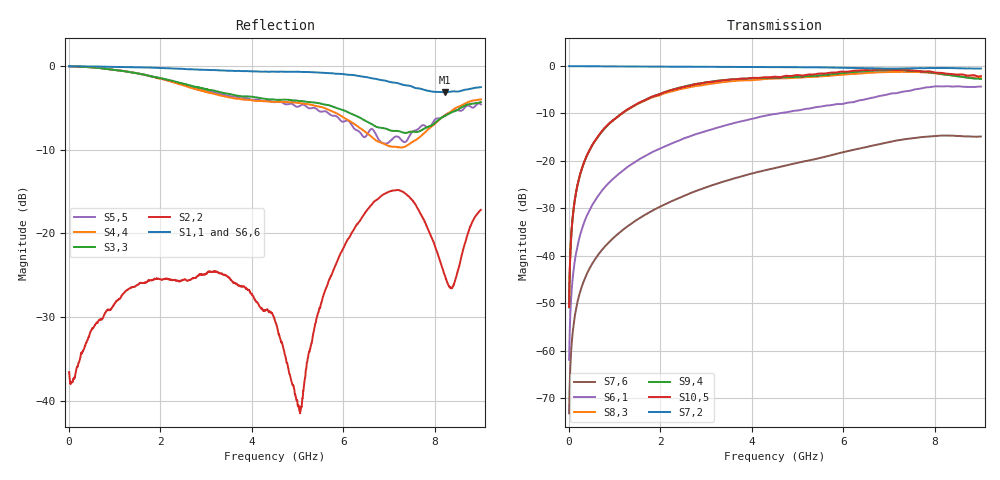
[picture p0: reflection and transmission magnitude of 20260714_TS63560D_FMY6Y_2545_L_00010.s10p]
# GHz S DB R 50
! CMT, SN0916, 25263762, 26.7.0
! Date: 15.07.2026 13:19:08
! Data: Format
! Freq S1.1:dB/Ang S1.2:dB/Ang S1.3:dB/Ang S1.4:dB/Ang S1.5:dB/Ang S1.6:dB/Ang S1.7:dB/Ang S1.8:dB/Ang S1.9:dB/Ang S1.10:dB/Ang
!  S2.1:dB/Ang S2.2:dB/Ang S2.3:dB/Ang S2.4:dB/Ang S2.5:dB/Ang S2.6:dB/Ang S2.7:dB/Ang S2.8:dB/Ang S2.9:dB/Ang S2.10:dB/Ang
!  S3.1:dB/Ang S3.2:dB/Ang S3.3:dB/Ang S3.4:dB/Ang S3.5:dB/Ang S3.6:dB/Ang S3.7:dB/Ang S3.8:dB/Ang S3.9:dB/Ang S3.10:dB/Ang
!  S4.1:dB/Ang S4.2:dB/Ang S4.3:dB/Ang S4.4:dB/Ang S4.5:dB/Ang S4.6:dB/Ang S4.7:dB/Ang S4.8:dB/Ang S4.9:dB/Ang S4.10:dB/Ang
!  S5.1:dB/Ang S5.2:dB/Ang S5.3:dB/Ang S5.4:dB/Ang S5.5:dB/Ang S5.6:dB/Ang S5.7:dB/Ang S5.8:dB/Ang S5.9:dB/Ang S5.10:dB/Ang
!  S6.1:dB/Ang S6.2:dB/Ang S6.3:dB/Ang S6.4:dB/Ang S6.5:dB/Ang S6.6:dB/Ang S6.7:dB/Ang S6.8:dB/Ang S6.9:dB/Ang S6.10:dB/Ang
!  S7.1:dB/Ang S7.2:dB/Ang S7.3:dB/Ang S7.4:dB/Ang S7.5:dB/Ang S7.6:dB/Ang S7.7:dB/Ang S7.8:dB/Ang S7.9:dB/Ang S7.10:dB/Ang
!  S8.1:dB/Ang S8.2:dB/Ang S8.3:dB/Ang S8.4:dB/Ang S8.5:dB/Ang S8.6:dB/Ang S8.7:dB/Ang S8.8:dB/Ang S8.9:dB/Ang S8.10:dB/Ang
!  S9.1:dB/Ang S9.2:dB/Ang S9.3:dB/Ang S9.4:dB/Ang S9.5:dB/Ang S9.6:dB/Ang S9.7:dB/Ang S9.8:dB/Ang S9.9:dB/Ang S9.10:dB/Ang
!  S10.1:dB/Ang S10.2:dB/Ang S10.3:dB/Ang S10.4:dB/Ang S10.5:dB/Ang S10.6:dB/Ang S10.7:dB/Ang S10.8:dB/Ang S10.9:dB/Ang S10.10:dB/Ang
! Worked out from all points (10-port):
!   2001 points, 10 MHz to 9 GHz, reference 50 ohm
!   strongest paths, dB at 10 MHz, 2.257 GHz, 4.505 GHz, 6.753 GHz, 9 GHz:
!     S7,2: -0.1, -0.2, -0.3, -0.6, -0.6
!     S10,5: -50.8, -5.1, -2.3, -0.8, -2.2
!     S9,4: -50.9, -5.1, -2.5, -1.0, -2.8
!     S8,3: -50.7, -5.4, -2.7, -1.4, -2.6
!     S6,1: -61.9, -16.4, -10.2, -6.5, -4.4
!     S7,6: -73.2, -28.5, -21.6, -16.6, -14.9
!   lowest |S11| = -3.1 dB at 8.213 GHz (marker M1), VSWR 5.60, Z = 11 - j23.7 ohm
!   |S11| at or under -10 dB: nowhere
